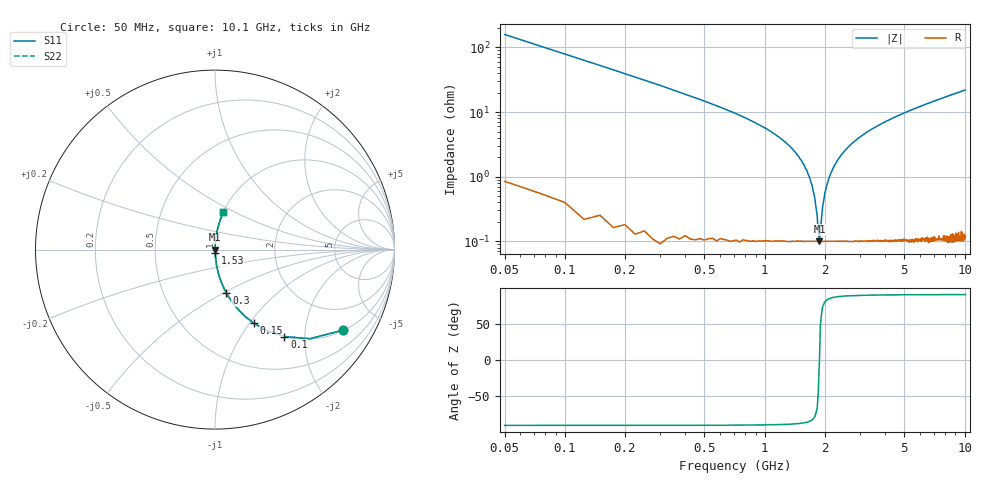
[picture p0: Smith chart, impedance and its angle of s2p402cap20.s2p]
! AVX Thin Film Operation		Date: April 2003
! Description: Accu-P® Series, Thin Film, SMD, RF Capacitor
! Part Number: 0402ZK200FBW
! 50 MHz  -  10.05 GHz
! Serial Measurements
# hz S db R 50
!	S11		S21		S12		S22
!	dB	Phase	dB	Phase	dB	Phase	dB	Phase
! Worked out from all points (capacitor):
!   400 points, 50 MHz to 10.1 GHz, reference 50 ohm
!   read as one part in series: C = 20 pF near 100 MHz
!   lowest |Z| = 100 mohm at 1.88 GHz (marker M1)
!   series resonance near 1.881 GHz, so ESL is about 360 pH
!   S11 on the Smith chart (normalised r, x): 50 MHz: 1.02, -3.18; 100 MHz: 1.01, -1.59; 150 MHz: 1.00, -1.05; 300 MHz: 1.00, -0.52; 1.53 GHz: 1.00, -0.04; 10.1 GHz: 1.00, +0.44
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5e7  -1.47 -32.1  -5.50 57.6  -5.50 57.6  -1.47 -32.1
1e8  -4.15 -51.4  -2.14 38.3  -2.14 38.3  -4.15 -51.4
1.5e8  -6.64 -62.0  -1.08 27.7  -1.08 27.7  -6.64 -62.0
3e8  -12.00 -75.3  -0.29 14.5  -0.29 14.5  -12.00 -75.3
6.75e8  -19.80 -83.6  -0.05 5.8  -0.05 5.8  -19.80 -83.6
1.18e9  -27.70 -86.2  -0.02 2.4  -0.02 2.4  -27.70 -86.2
1.53e9  -35.00 -85.7  -0.01 1.0  -0.01 1.0  -35.00 -85.7
1.73e9  -42.90 -81.6  -0.01 0.4  -0.01 0.4  -42.90 -81.6
1.78e9  -46.40 -77.7  -0.01 0.3  -0.01 0.3  -46.40 -77.7
1.83e9  -51.90 -66.6  -0.01 0.1  -0.01 0.1  -51.90 -66.6
1.85e9  -56.30 -49.4  -0.01 0.1  -0.01 0.1  -56.30 -49.4
1.88e9  -60.00 -1.7  -0.01 0.0  -0.01 0.0  -60.00 -1.7
1.95e9  -49.30 72.9  -0.01 -0.2  -0.01 -0.2  -49.30 72.9
2e9  -45.10 79.3  -0.01 -0.3  -0.01 -0.3  -45.10 79.3
2.1e9  -40.30 83.5  -0.01 -0.6  -0.01 -0.6  -40.30 83.5
2.2e9  -37.30 85.0  -0.01 -0.8  -0.01 -0.8  -37.30 85.0
2.7e9  -30.00 86.4  -0.01 -1.8  -0.01 -1.8  -30.00 86.4
3.4e9  -25.50 85.9  -0.02 -3.1  -0.02 -3.1  -25.50 85.9
5.08e9  -20.10 83.7  -0.05 -5.7  -0.05 -5.7  -20.10 83.7
6.75e9  -17.10 81.6  -0.09 -8.0  -0.09 -8.0  -17.10 81.6
8.43e9  -15.00 79.4  -0.15 -10.3  -0.15 -10.3  -15.00 79.4
1.01e10  -13.40 77.3  -0.21 -12.4  -0.21 -12.4  -13.40 77.3
